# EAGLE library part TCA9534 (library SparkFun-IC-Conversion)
Texas Instruments TCA9534 I2C -> GPIO Expander This I2C -> GPIO Expander allows you to attach 8 GPIO to your I2C bus. With 8 different addresses, up to 64 GPIO are possible on one I2C bus
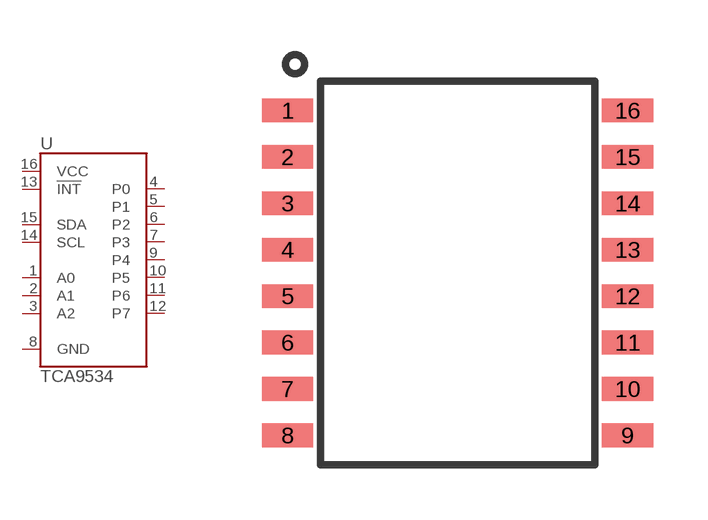
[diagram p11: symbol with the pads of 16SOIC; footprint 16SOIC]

Designator prefix U

## TCA9534U (PROD_ID: IC-14889; VALUE: TCA9534)  [16SOIC]
1  A0
2  A1
3  A2
4  P0
5  P1
6  P2
7  P3
8  GND
9  P4
10  P5
11  P6
12  P7
13  !INT
14  SCL
15  SDA
16  VCC

## Footprint 16SOIC (pad centres in mm)
smd 1.397 x 0.648: 1 -4.65,4.445; 2 -4.65,3.175; 3 -4.65,1.905; 4 -4.65,0.635; 5 -4.65,-0.635; 6 -4.65,-1.905; 7 -4.65,-3.175; 8 -4.65,-4.445; 9 4.65,-4.445; 10 4.65,-3.175; 11 4.65,-1.905; 12 4.65,-0.635; 13 4.65,0.635; 14 4.65,1.905; 15 4.65,3.175; 16 4.65,4.445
